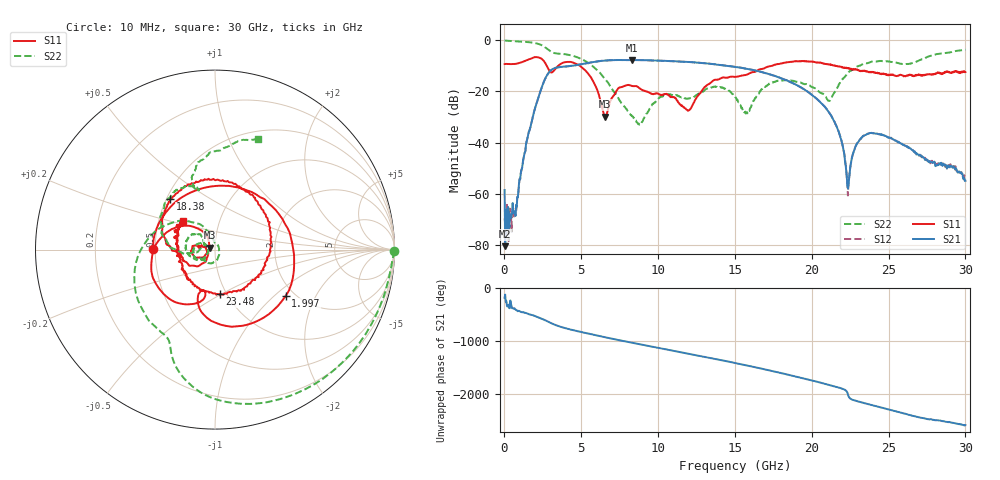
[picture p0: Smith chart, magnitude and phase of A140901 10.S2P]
!  2-Port S-parameters saved by WinCal
! VAR MeasName=S-Parameters (CALIBRATED_DATA) read from VNA (N5244A)
! VAR MeasDate=11/3/2014 9:27:33 AM
! VAR NAME=A140901 10
! VAR FILENAME=A140901 10.S2P
! VAR DATE=11/3/2014 9:27:33 AM
! VAR PHYS_PORTS=1,2
# Hz S RI R 50
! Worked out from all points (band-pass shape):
!   801 points, 10 MHz to 30 GHz, reference 50 ohm
!   highest |S21| = -7.66 dB at 8.295 GHz (marker M1); lowest = -80.6 dB at 47.49 MHz (marker M2)
!   |S21| within 3 dB of the highest: 3.384 GHz to 15.34 GHz (11.95 GHz wide, 128 % of centre)
!   lowest |S11| = -29.8 dB at 6.533 GHz (marker M3), VSWR 1.07, Z = 47 + j0.959 ohm
!   |S11| at or under -10 dB: 2.758 GHz to 3.487 GHz (729.7 MHz wide, 23.4 % of centre); 4.924 GHz to 17.36 GHz (12.44 GHz wide, 112 % of centre); 21.64 GHz to end of sweep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
!   |S22| runs from -33.0 to 0.0 dB; largest |S21 - S12| = 0.0026
!   S11 on the Smith chart (normalised r, x): 10 MHz: 0.49, +0.01; 1.997 GHz: 1.79, -1.19; 18.38 GHz: 0.53, +0.34; 23.48 GHz: 0.93, -0.49; 30 GHz: 0.67, +0.23
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1e7  -0.3435 0.00604  -0.00117 -5.85e-05  -0.000141 0.000297  0.9981 -0.00784
4.74875e7  -0.3447 0.0294  -4.09e-05 -8.41e-05  3.36e-05 -0.000252  0.9931 -0.0372
7.222625e8  -0.0905 0.3357  0.000265 -0.00025  0.000495 -0.000193  0.8612 -0.4335
1.996838e9  0.3936 -0.2586  -0.0457 -0.0117  -0.0458 -0.0116  0.2185 -0.8587
3.009e9  -0.0731 -0.2269  0.1111 0.2324  0.1107 0.2322  -0.2469 -0.5567
3.75875e9  -0.2007 -0.299  0.2889 -0.0946  0.2885 -0.0947  -0.3394 -0.4231
5.033325e9  -0.2867 0.0805  -0.1215 -0.3205  -0.1215 -0.3201  -0.4275 -0.0334
6.532825e9  -0.0306 0.0102  -0.3599 0.18  -0.3597 0.18  -0.1 0.1463
8.294738e9  -0.1286 0.00271  0.2759 0.3089  0.2755 0.3082  0.00704 0.032
8.85705e9  -0.1092 0.0233  0.3967 0.1129  0.3961 0.1125  0.0235 -0.00289
1.001916e10  -0.0897 0.0109  0.2614 -0.3073  0.2605 -0.307  -0.0102 -0.072
1.23059e10  -0.0425 -0.041  -0.3726 -0.00952  -0.3733 -0.00949  -0.0596 -0.0508
1.365545e10  -0.1412 -0.0896  -0.0782 0.3321  -0.0779 0.3332  -0.1192 -0.0342
1.5005e10  -0.1912 -0.0291  0.2776 0.1226  0.2777 0.1217  -0.069 0.0351
1.579224e10  -0.2135 -0.014  0.2526 -0.1157  0.2521 -0.1163  -0.0381 -0.00935
1.837888e10  -0.248 0.2805  -0.1596 0.0399  -0.1594 0.0399  -0.159 0.0475
2.002832e10  0.0952 0.3736  0.0551 0.0648  0.0546 0.0651  -0.0855 0.085
2.16028e10  0.3108 0.0458  0.00672 -0.0201  0.00671 -0.02  -0.1067 -0.0178
2.235255e10  0.2559 -0.1321  -0.00103 0.000719  -0.000636 0.000663  -0.2322 0.00653
2.347718e10  0.0253 -0.2485  0.0127 -0.00585  0.013 -0.00573  -0.3054 0.1853
2.501416e10  -0.1672 -0.1219  -0.0095 -0.00794  -0.00948 -0.00799  -0.1526 0.3567
3e10  -0.1787 0.16  0.000349 -0.00175  0.000479 -0.00172  0.2376 0.6167
